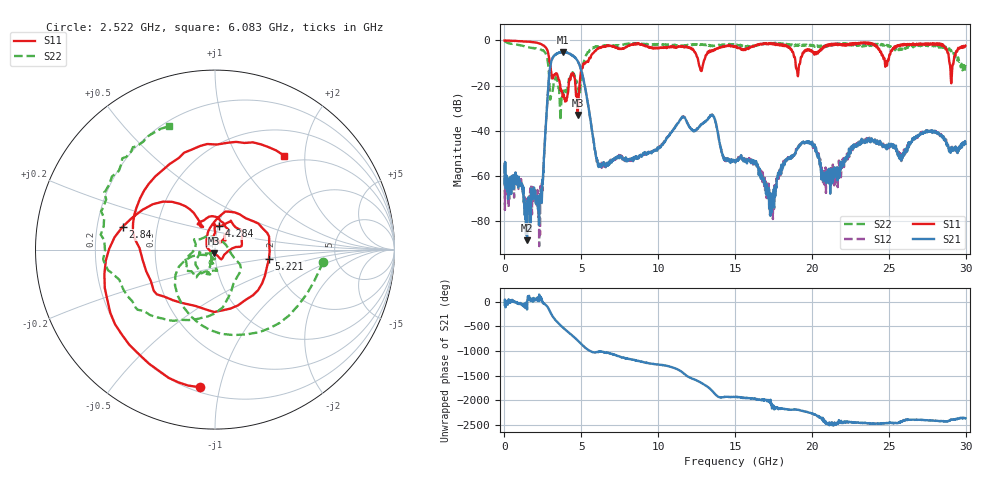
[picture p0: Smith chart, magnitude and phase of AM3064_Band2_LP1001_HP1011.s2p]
# Hz S DB R 50.0
!freq dBS11 angS11 dBS21 angS21 dBS12 angS12 dBS22 angS22
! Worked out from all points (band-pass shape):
!   1600 points, 10 MHz to 29.98 GHz, reference 50 ohm
!   highest |S21| = -5.13 dB at 3.777 GHz (marker M1); lowest = -88.6 dB at 1.472 GHz (marker M2)
!   |S21| within 3 dB of the highest: 3.116 GHz to 4.661 GHz (1.546 GHz wide, 39.8 % of centre)
!   lowest |S11| = -33.1 dB at 4.752 GHz (marker M3), VSWR 1.05, Z = 49.5 - j2.15 ohm
!   |S11| at or under -10 dB: 2.956 GHz to 5.261 GHz (2.305 GHz wide, 56.1 % of centre); 12.63 GHz to 12.94 GHz (310.1 MHz wide, 2.43 % of centre); 18.93 GHz to 19.23 GHz (294.7 MHz wide, 1.54 % of centre)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
!   |S22| runs from -35.4 to -0.3 dB; largest |S21 - S12| = 0.016
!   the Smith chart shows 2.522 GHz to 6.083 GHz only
!   S11 on the Smith chart (normalised r, x): 2.522 GHz: 0.23, -0.87; 2.84 GHz: 0.31, +0.11; 4.284 GHz: 1.01, +0.27; 5.221 GHz: 1.84, -0.21; 6.083 GHz: 0.88, +1.60
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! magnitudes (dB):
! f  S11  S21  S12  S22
! 10 MHz  -0.1  -54.7  -55.2  -0.3
! 1.472 GHz  -0.6  -88.6  -79.0  -3.0
! 2.259 GHz  -1.4  -81.1  -91.1  -3.7
! 2.522 GHz  -2.2  -58.0  -57.9  -4.4
! 2.84 GHz  -5.5  -21.5  -21.4  -10.5
! 3.777 GHz  -24.5  -5.1  -5.2  -26.0
! 4.284 GHz  -17.5  -6.2  -5.9  -16.4
! 4.752 GHz  -33.1  -9.1  -9.1  -20.8
! 5.015 GHz  -12.9  -13.8  -13.7  -15.0
! 5.221 GHz  -10.3  -20.0  -19.9  -8.3
! 6.083 GHz  -3.7  -55.4  -53.1  -2.7
! 10 GHz  -3.4  -47.7  -47.5  -1.8
! 13.49 GHz  -4.4  -33.1  -33.2  -2.3
! 15 GHz  -2.6  -53.5  -53.9  -1.9
! 16.35 GHz  -2.3  -54.4  -54.4  -2.5
! 17.39 GHz  -1.6  -68.0  -73.7  -1.3
! 18.27 GHz  -2.5  -53.9  -52.9  -1.9
! 19.99 GHz  -4.6  -45.9  -45.8  -2.0
! 21.21 GHz  -2.2  -58.0  -56.6  -2.0
! 25 GHz  -8.4  -45.7  -47.3  -2.2
! 29.08 GHz  -17.7  -48.0  -48.0  -5.2
! 29.98 GHz  -2.4  -45.8  -45.5  -10.9
